| TEXAS INSTRUMENTS INCORPORATED
| Standard Linear and Logic Group
| IBIS Model of SN74ALVCH162373
| 16-Bit Transparent D-type Latch wit 3 state outputs
| This file contains package information for the following:
|  SSOP 48-pin (DL) package as [Component] ALVCH162373_DL
|  VFBGA 48-pin (GQL) package as [Component] ALVCH162373_GQL
|  TSSOP 48-pin (DGG) package as [Component] ALVCH162373_DGG
| This device can be powered at the following Vccs:
|  1.8 volt Vcc
|  2.5 volt Vcc
|  3.3 volt Vcc
| This file provides unique models under the [Model Selector] for each Vcc.
| For operation at a specific Vcc, select the appropriate model after each
| [Model Selector] keyword.
[IBIS Ver]   3.2
[Comment char]  |_char
[File Name]   sn74alvch162373.ibs
[File Rev]   1.1 | B_die
[Date]   March 21, 2005
[Source]   Data created from TI-SPICE simulations at TI-SLL.
[Notes]   The following is an IBIS list for the ALVCH162373.
   Please contact sllibis@ti.com with questions and
   comments concerning SLL IBIS models.
   This IBIS model is created from a BA (back annotated netlist)
   - FILE REV HISTORY
   - 1.1 Release IBIS file on 03/28/05
   - Non-monotonic data in ground-clamp due to bus-hold
   - Non-monotonic data in pullup and pulldown data due to
   resistor at output.
[Disclaimer] Property of Texas Instruments Incorporated.  Unauthorized
   reproduction and/or distribution is strictly prohibited.
   This product is protected under copyright law.
   Created  2005, (C) Copyright  2005, Texas Instruments
   Incorporated, All Rights Reserved
   UNLESS THERE IS A SIGNED, WRITTEN AGREEMENT TO THE
   CONTRARY, TEXAS INSTRUMENTS (TI) IS PROVIDING THE IBIS
   MODELS  AND WITHOUT ANY WARRANTY, EXPRESSED OR
   IMPLIED.  TI assumes no liability for:
   1) the accuracy of the IBIS models provided to your
   company;
   2) the proper functioning of these IBIS Models in your
   design or for any resulting applications; or
   3) infringement of patents, copyrights or intellectual
   property rights resulting from your use of these IBIS
   models.
   TI provides IBIS Models as a service to our customers.
   You and your company shall not distribute, sell or give
   these models to anyone else without prior written
   permission from TI.
   TI reserves the right to make changes to our products or
   to discontinue any semiconductor product or service
   without notice, and advises our customers to obtain the
   latest version of relevant information to verify, before
   placing orders, that the information being relied on is
   current.
   Please be aware that your receipt and use of the IBIS
   information provided shall serve as acceptance of these
   terms and conditions.  If you do not accept these terms,
   you should return or destroy the IBIS models and any
   other accompanying information immediately.
| Component ALVCH162373_DL 48-pin SSOP
[Component]   ALVCH162373_DL
[Manufacturer]   Texas Instruments, Inc.
[Package]
|   typ   min   max
R_pkg   4.800e-02   3.800e-02   5.300e-02
L_pkg   6.046e-09   5.084e-09   7.968e-09
C_pkg   8.130e-13   5.690e-13   1.157e-12
[Pin]   signal_name   model_name   R_pin   L_pin   C_pin
1   1NOE   ALVCH162373_OE   4.600e-02   7.968e-09   1.017e-12
2   1Q1   ALVCH162373_OUT   4.400e-02   7.299e-09   1.157e-12
3   1Q2   ALVCH162373_OUT   4.300e-02   6.765e-09   1.058e-12
4   GND   GND   4.100e-02   6.269e-09   9.330e-13
5   1Q3   ALVCH162373_OUT   3.800e-02   5.856e-09   8.290e-13
6   1Q4   ALVCH162373_OUT   4.600e-02   5.802e-09   7.900e-13
7   VCC   POWER   5.000e-02   5.656e-09   7.380e-13
8   1Q5   ALVCH162373_OUT   5.300e-02   5.500e-09   6.430e-13
9   1Q6   ALVCH162373_OUT   5.200e-02   5.304e-09   6.060e-13
10   GND   GND   5.300e-02   5.189e-09   5.830e-13
11   1Q7   ALVCH162373_OUT   5.100e-02   5.084e-09   5.690e-13
12   1Q8   ALVCH162373_OUT   5.300e-02   5.862e-09   8.330e-13
13   2Q1   ALVCH162373_OUT   5.300e-02   5.862e-09   8.330e-13
14   2Q2   ALVCH162373_OUT   5.100e-02   5.084e-09   5.690e-13
15   GND   GND   5.300e-02   5.189e-09   5.830e-13
16   2Q3   ALVCH162373_OUT   5.200e-02   5.304e-09   6.060e-13
17   2Q4   ALVCH162373_OUT   5.300e-02   5.500e-09   6.430e-13
18   VCC   POWER   5.000e-02   5.656e-09   7.380e-13
19   2Q5   ALVCH162373_OUT   4.600e-02   5.802e-09   7.900e-13
20   2Q6   ALVCH162373_OUT   3.800e-02   5.856e-09   8.290e-13
21   GND   GND   4.100e-02   6.269e-09   9.330e-13
22   2Q7   ALVCH162373_OUT   4.300e-02   6.765e-09   1.058e-12
23   2Q8   ALVCH162373_OUT   4.400e-02   7.299e-09   1.157e-12
24   2NOE   ALVCH162373_OE   4.600e-02   7.968e-09   1.017e-12
25   2LE   ALVCH162373_LE   4.600e-02   7.968e-09   1.017e-12
26   2D8   ALVCH162373_IN   4.400e-02   7.299e-09   1.157e-12
27   2D7   ALVCH162373_IN   4.300e-02   6.765e-09   1.058e-12
28   GND   GND   4.100e-02   6.269e-09   9.330e-13
29   2D6   ALVCH162373_IN   3.800e-02   5.856e-09   8.290e-13
30   2D5   ALVCH162373_IN   4.600e-02   5.802e-09   7.900e-13
31   VCC   POWER   5.000e-02   5.656e-09   7.380e-13
32   2D4   ALVCH162373_IN   5.300e-02   5.500e-09   6.430e-13
33   2D3   ALVCH162373_IN   5.200e-02   5.304e-09   6.060e-13
34   GND   GND   5.300e-02   5.189e-09   5.830e-13
35   2D2   ALVCH162373_IN   5.100e-02   5.084e-09   5.690e-13
36   2D1   ALVCH162373_IN   5.300e-02   5.862e-09   8.330e-13
37   1D8   ALVCH162373_IN   5.300e-02   5.862e-09   8.330e-13
38   1D7   ALVCH162373_IN   5.100e-02   5.084e-09   5.690e-13
39   GND   GND   5.300e-02   5.189e-09   5.830e-13
40   1D6   ALVCH162373_IN   5.200e-02   5.304e-09   6.060e-13
41   1D5   ALVCH162373_IN   5.300e-02   5.500e-09   6.430e-13
42   VCC   POWER   5.000e-02   5.656e-09   7.380e-13
43   1D4   ALVCH162373_IN   4.600e-02   5.802e-09   7.900e-13
44   1D3   ALVCH162373_IN   3.800e-02   5.856e-09   8.290e-13
45   GND   GND   4.100e-02   6.269e-09   9.330e-13
46   1D2   ALVCH162373_IN   4.300e-02   6.765e-09   1.058e-12
47   1D1   ALVCH162373_IN   4.400e-02   7.299e-09   1.157e-12
48   1LE   ALVCH162373_LE   4.600e-02   7.967e-09   1.017e-12
| Component ALVCH162373_GQL 48-pin VFBGA
[Component]   ALVCH162373_GQL
[Manufacturer]   Texas Instruments, Inc.
[Package]
|   typ   min   max
R_pkg   7.900e-02   4.500e-02   9.400e-02
L_pkg   2.264e-09   1.398e-09   2.722e-09
C_pkg   3.060e-13   1.170e-13   4.040e-13
[Pin]   signal_name   model_name   R_pin   L_pin   C_pin
A1   1NOE   ALVCH162373_OE   5.100e-02   1.531e-09   2.100e-13
B2   1Q1   ALVCH162373_OUT   7.300e-02   2.572e-09   3.120e-13
B1   1Q2   ALVCH162373_OUT   7.100e-02   1.835e-09   2.320e-13
B3   GND   GND   9.400e-02   2.717e-09   3.830e-13
C2   1Q3   ALVCH162373_OUT   8.900e-02   2.534e-09   3.500e-13
C1   1Q4   ALVCH162373_OUT   7.100e-02   1.831e-09   2.310e-13
C3   VCC   POWER   9.400e-02   2.722e-09   3.920e-13
D2   1Q5   ALVCH162373_OUT   9.000e-02   2.551e-09   3.520e-13
D1   1Q6   ALVCH162373_OUT   7.200e-02   1.846e-09   2.440e-13
D3   GND   GND   9.400e-02   2.719e-09   4.030e-13
E2   1Q7   ALVCH162373_OUT   8.900e-02   2.541e-09   3.510e-13
E1   1Q8   ALVCH162373_OUT   7.200e-02   1.850e-09   2.270e-13
F1   2Q1   ALVCH162373_OUT   7.200e-02   1.850e-09   2.270e-13
F2   2Q2   ALVCH162373_OUT   8.900e-02   2.541e-09   3.510e-13
G3   GND   GND   9.400e-02   2.718e-09   4.040e-13
G1   2Q3   ALVCH162373_OUT   7.200e-02   1.847e-09   2.440e-13
G2   2Q4   ALVCH162373_OUT   9.000e-02   2.551e-09   3.520e-13
H3   VCC   POWER   9.400e-02   2.721e-09   3.920e-13
H1   2Q5   ALVCH162373_OUT   7.000e-02   1.830e-09   2.310e-13
H2   2Q6   ALVCH162373_OUT   8.800e-02   2.524e-09   3.500e-13
J3   GND   GND   9.300e-02   2.709e-09   3.820e-13
J1   2Q7   ALVCH162373_OUT   7.100e-02   1.851e-09   2.330e-13
J2   2Q8   ALVCH162373_OUT   5.600e-02   2.605e-09   3.900e-13
K1   2NOE   ALVCH162373_OE   4.500e-02   1.398e-09   1.170e-13
K6   2LE   ALVCH162373_LE   4.500e-02   1.512e-09   1.930e-13
J5   2D8   ALVCH162373_IN   5.500e-02   2.492e-09   3.130e-13
J6   2D7   ALVCH162373_IN   7.000e-02   1.821e-09   2.300e-13
J4   GND   GND   9.300e-02   2.703e-09   3.820e-13
H5   2D6   ALVCH162373_IN   8.900e-02   2.529e-09   3.500e-13
H6   2D5   ALVCH162373_IN   7.100e-02   1.826e-09   2.300e-13
H4   VCC   POWER   9.400e-02   2.722e-09   3.910e-13
G5   2D4   ALVCH162373_IN   9.000e-02   2.551e-09   3.520e-13
G6   2D3   ALVCH162373_IN   7.200e-02   1.846e-09   2.440e-13
G4   GND   GND   9.400e-02   2.719e-09   4.040e-13
F5   2D2   ALVCH162373_IN   8.800e-02   2.510e-09   3.490e-13
F6   2D1   ALVCH162373_IN   7.200e-02   1.850e-09   2.270e-13
E6   1D8   ALVCH162373_IN   7.100e-02   1.850e-09   2.270e-13
E5   1D7   ALVCH162373_IN   8.900e-02   2.529e-09   3.500e-13
D4   GND   GND   9.400e-02   2.719e-09   4.030e-13
D6   1D6   ALVCH162373_IN   7.200e-02   1.847e-09   2.430e-13
D5   1D5   ALVCH162373_IN   8.900e-02   2.550e-09   3.520e-13
C4   VCC   POWER   9.400e-02   2.722e-09   3.910e-13
C6   1D4   ALVCH162373_IN   7.100e-02   1.827e-09   2.300e-13
C5   1D3   ALVCH162373_IN   8.900e-02   2.539e-09   3.500e-13
B4   GND   GND   9.300e-02   2.705e-09   3.820e-13
B6   1D2   ALVCH162373_IN   7.100e-02   1.831e-09   2.270e-13
B5   1D1   ALVCH162373_IN   7.300e-02   2.685e-09   3.800e-13
A6   1LE   ALVCH162373_LE   5.100e-02   1.417e-09   1.330e-13
| Component ALVCH162373_DGG 48-pin TSSOP
[Component]   ALVCH162373_DGG
[Manufacturer]   Texas Instruments, Inc.
[Package]
|   typ   min   max
R_pkg   4.400e-02   3.800e-02   5.100e-02
L_pkg   3.019e-09   2.486e-09   4.099e-09
C_pkg   5.070e-13   3.340e-13   8.090e-13
[Pin]   signal_name   model_name   R_pin   L_pin   C_pin
1   1NOE   ALVCH162373_OE   4.100e-02   4.017e-09   7.590e-13
2   1Q1   ALVCH162373_OUT   4.200e-02   3.737e-09   7.920e-13
3   1Q2   ALVCH162373_OUT   4.200e-02   3.480e-09   6.610e-13
4   GND   GND   3.800e-02   3.131e-09   5.750e-13
5   1Q3   ALVCH162373_OUT   4.700e-02   3.122e-09   5.660e-13
6   1Q4   ALVCH162373_OUT   4.300e-02   2.948e-09   5.040e-13
7   VCC   POWER   4.500e-02   2.845e-09   3.970e-13
8   1Q5   ALVCH162373_OUT   4.900e-02   2.835e-09   3.940e-13
9   1Q6   ALVCH162373_OUT   4.800e-02   2.715e-09   3.780e-13
10   GND   GND   5.000e-02   2.664e-09   3.630e-13
11   1Q7   ALVCH162373_OUT   5.000e-02   2.585e-09   3.480e-13
12   1Q8   ALVCH162373_OUT   4.900e-02   2.550e-09   3.370e-13
13   2Q1   ALVCH162373_OUT   4.900e-02   2.541e-09   3.360e-13
14   2Q2   ALVCH162373_OUT   5.000e-02   2.574e-09   3.480e-13
15   GND   GND   4.900e-02   2.618e-09   3.590e-13
16   2Q3   ALVCH162373_OUT   4.600e-02   2.671e-09   3.750e-13
17   2Q4   ALVCH162373_OUT   4.500e-02   2.754e-09   3.890e-13
18   VCC   POWER   4.400e-02   2.823e-09   4.500e-13
19   2Q5   ALVCH162373_OUT   4.200e-02   2.968e-09   5.030e-13
20   2Q6   ALVCH162373_OUT   5.100e-02   3.108e-09   5.350e-13
21   GND   GND   4.200e-02   3.175e-09   5.870e-13
22   2Q7   ALVCH162373_OUT   4.100e-02   3.449e-09   6.780e-13
23   2Q8   ALVCH162373_OUT   4.400e-02   3.766e-09   8.040e-13
24   2NOE   ALVCH162373_OE   4.300e-02   4.065e-09   7.610e-13
25   2LE   ALVCH162373_LE   4.100e-02   3.994e-09   7.570e-13
26   2D8   ALVCH162373_IN   3.900e-02   3.649e-09   7.890e-13
27   2D7   ALVCH162373_IN   3.800e-02   3.362e-09   6.600e-13
28   GND   GND   3.800e-02   3.082e-09   5.740e-13
29   2D6   ALVCH162373_IN   4.400e-02   2.990e-09   5.220e-13
30   2D5   ALVCH162373_IN   4.100e-02   2.917e-09   4.950e-13
31   VCC   POWER   4.300e-02   2.820e-09   4.480e-13
32   2D4   ALVCH162373_IN   4.300e-02   2.699e-09   3.850e-13
33   2D3   ALVCH162373_IN   4.500e-02   2.628e-09   3.720e-13
34   GND   GND   4.600e-02   2.556e-09   3.560e-13
35   2D2   ALVCH162373_IN   4.600e-02   2.495e-09   3.440e-13
36   2D1   ALVCH162373_IN   4.700e-02   2.487e-09   3.340e-13
37   1D8   ALVCH162373_IN   4.700e-02   2.490e-09   3.350e-13
38   1D7   ALVCH162373_IN   4.600e-02   2.486e-09   3.430e-13
39   GND   GND   4.500e-02   2.566e-09   3.560e-13
40   1D6   ALVCH162373_IN   4.400e-02   2.639e-09   3.740e-13
41   1D5   ALVCH162373_IN   4.300e-02   2.701e-09   3.860e-13
42   VCC   POWER   4.300e-02   2.817e-09   4.500e-13
43   1D4   ALVCH162373_IN   4.100e-02   2.935e-09   5.010e-13
44   1D3   ALVCH162373_IN   4.700e-02   3.035e-09   5.290e-13
45   GND   GND   4.300e-02   3.171e-09   5.890e-13
46   1D2   ALVCH162373_IN   4.000e-02   3.415e-09   6.820e-13
47   1D1   ALVCH162373_IN   4.300e-02   3.741e-09   8.090e-13
48   1LE   ALVCH162373_LE   4.400e-02   4.099e-09   7.640e-13
| Model ALVCH162373_LE
[Model Selector]   ALVCH162373_LE
ALVCH162373_LE_18   1.8 volt Vcc
ALVCH162373_LE_25   2.5 volt Vcc
ALVCH162373_LE_33   3.3 volt Vcc
| Model ALVCH162373_IN
[Model Selector]   ALVCH162373_IN
ALVCH162373_IN_18   1.8 volt Vcc
ALVCH162373_IN_25   2.5 volt Vcc
ALVCH162373_IN_33   3.3 volt Vcc
| Model ALVCH162373_OE
[Model Selector]   ALVCH162373_OE
ALVCH162373_OE_18   1.8 volt Vcc
ALVCH162373_OE_25   2.5 volt Vcc
ALVCH162373_OE_33   3.3 volt Vcc
| Model ALVCH162373_OUT
[Model Selector]   ALVCH162373_OUT
ALVCH162373_OUT_18   1.8 volt Vcc
ALVCH162373_OUT_25   2.5 volt Vcc
ALVCH162373_OUT_33   3.3 volt Vcc
| Models and submodels in the file (12): ALVCH162373_LE_18 (Input), ALVCH162373_LE_25 (Input), ALVCH162373_LE_33 (Input), ALVCH162373_IN_18 (Input), ALVCH162373_IN_25 (Input), ALVCH162373_IN_33 (Input), ALVCH162373_OE_18 (Input), ALVCH162373_OE_25 (Input), ALVCH162373_OE_33 (Input), ALVCH162373_OUT_18 (3-state), ALVCH162373_OUT_25 (3-state), ALVCH162373_OUT_33 (3-state)
